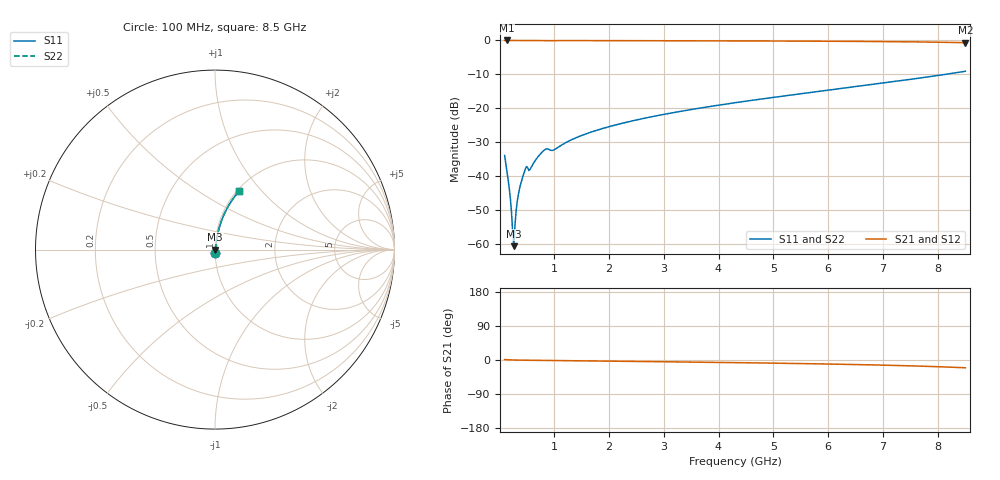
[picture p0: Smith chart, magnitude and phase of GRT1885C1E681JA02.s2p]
!Murata Part Number: GRT1885C1E681JA02
!These Parameters are Measured in Series Mode Connection
!Data Generated on Jun 19, 2026
!  o--ll--o
!Port1  Port2
!  o------o
!Operation Temp=25[degC], DC Bias Voltage=0[V]
!Freq. Start=100[MHz] Stop=9[GHz] 401[Steps]
# Hz S RI R 50
!Freq.(Hz) S11(Real) S11(Imag) S21(Real) S21(Imag) S12(Real) S12(Imag) S22(Real) S22(Imag)
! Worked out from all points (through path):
!   401 points, 100 MHz to 8.5 GHz, reference 50 ohm
!   highest |S21| = -0.01 dB at 142 MHz (marker M1); lowest = -0.7 dB at 8.5 GHz (marker M2)
!   group delay of S21, straight-line fit = 6.1 ps
!   lowest |S11| = -60.8 dB at 268 MHz (marker M3), VSWR 1.00, Z = 50.1 + j0.0239 ohm
!   |S11| at or under -10 dB: start of sweep to 8.142 GHz
!   |S22| runs from -60.8 to -9.1 dB; largest |S21 - S12| = 0
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1e8  0.000955 -0.02  0.999 0.02  0.999 0.02  0.000955 -0.02
1.42e8  0.000745 -0.0117  0.9993 0.0117  0.9993 0.0117  0.000745 -0.0117
1.84e8  0.000724 -0.00657  0.9993 0.00657  0.9993 0.00657  0.000724 -0.00657
2.26e8  0.000781 -0.0028  0.9992 0.0028  0.9992 0.0028  0.000781 -0.0028
2.47e8  0.000828 -0.00121  0.9992 0.00121  0.9992 0.00121  0.000828 -0.00121
2.68e8  0.000885 0.000238  0.9991 -0.000238  0.9991 -0.000238  0.000885 0.000238
2.89e8  0.000952 0.00159  0.999 -0.00159  0.999 -0.00159  0.000952 0.00159
3.1e8  0.00103 0.00286  0.999 -0.00286  0.999 -0.00286  0.00103 0.00286
3.31e8  0.00112 0.00407  0.9989 -0.00407  0.9989 -0.00407  0.00112 0.00407
3.73e8  0.00134 0.00638  0.9987 -0.00638  0.9987 -0.00638  0.00134 0.00638
4.36e8  0.00193 0.0098  0.9981 -0.0098  0.9981 -0.0098  0.00193 0.0098
4.78e8  0.00312 0.0122  0.9969 -0.0122  0.9969 -0.0122  0.00312 0.0122
5.83e8  0.0031 0.013  0.9969 -0.013  0.9969 -0.013  0.0031 0.013
8.35e8  0.00656 0.0235  0.9934 -0.0235  0.9934 -0.0235  0.00656 0.0235
1.003e9  0.00652 0.0234  0.9935 -0.0234  0.9935 -0.0234  0.00652 0.0234
1.507e9  0.00639 0.039  0.9936 -0.039  0.9936 -0.039  0.00639 0.039
2.116e9  0.00898 0.0556  0.991 -0.0556  0.991 -0.0556  0.00898 0.0556
2.914e9  0.013 0.0774  0.987 -0.0774  0.987 -0.0774  0.013 0.0774
4.3e9  0.0226 0.1181  0.9774 -0.1181  0.9774 -0.1181  0.0226 0.1181
5.707e9  0.0387 0.1672  0.9613 -0.1672  0.9613 -0.1672  0.0387 0.1672
7.114e9  0.0682 0.2315  0.9318 -0.2315  0.9318 -0.2315  0.0682 0.2315
8.5e9  0.133 0.3245  0.867 -0.3245  0.867 -0.3245  0.133 0.3245
